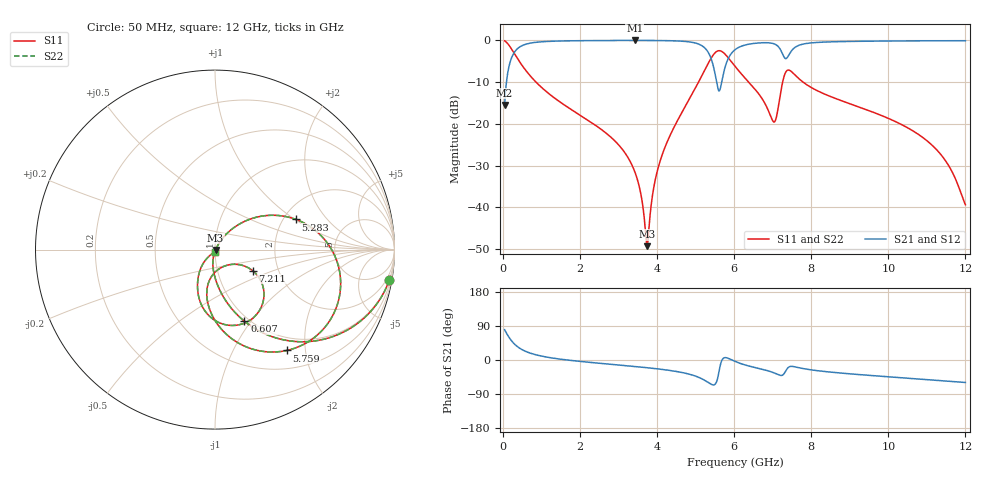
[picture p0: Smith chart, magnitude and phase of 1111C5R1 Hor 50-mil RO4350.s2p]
# GHz S MA R 50
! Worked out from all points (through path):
!   11951 points, 50 MHz to 12 GHz, reference 50 ohm
!   highest |S21| = -0.03 dB at 3.427 GHz (marker M1); lowest = -15.5 dB at 50 MHz (marker M2)
!   group delay of S21, straight-line fit = 16.3 ps
!   lowest |S11| = -49.3 dB at 3.745 GHz (marker M3), VSWR 1.01, Z = 50.3 - j0.136 ohm
!   |S11| at or under -10 dB: 864.7 MHz to 5.079 GHz (4.215 GHz wide, 142 % of centre); 6.381 GHz to 7.26 GHz (879.6 MHz wide, 12.9 % of centre); 7.79 GHz to end of sweep
!   |S22| runs from -49.3 to -0.1 dB; largest |S21 - S12| = 0
!   S11 on the Smith chart (normalised r, x): 50 MHz: 1, -11; 607 MHz: 0.95, -0.93; 5.283 GHz: 2.33, +1.02; 5.759 GHz: 0.78, -1.66; 7.211 GHz: 1.48, -0.37; 12 GHz: 1.00, -0.02
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0.05  0.9858 -10.0  0.1681 80.0  0.1681 80.0  0.9858 -10.0
0.238  0.7759 -40.4  0.6304 49.6  0.6304 49.6  0.7759 -40.4
0.607  0.432 -67.6  0.9011 22.3  0.9011 22.3  0.432 -67.6
2.042  0.1242 -93.4  0.9908 -4.1  0.9908 -4.1  0.1242 -93.4
2.956  0.05945 -100.9  0.9961 -12.7  0.9961 -12.7  0.05945 -100.9
3.427  0.02665 -101.5  0.9968 -17.1  0.9968 -17.1  0.02665 -101.5
3.579  0.01485 -97.2  0.9967 -18.6  0.9967 -18.6  0.01485 -97.2
3.745  0.003438 -23.2  0.9963 -20.3  0.9963 -20.3  0.003438 -23.2
4.034  0.03005 57.3  0.9946 -23.6  0.9946 -23.6  0.03005 57.3
4.844  0.1993 46.1  0.9579 -37.5  0.9579 -37.5  0.1993 46.1
5.283  0.4817 20.4  0.7726 -56.4  0.7726 -56.4  0.4817 20.4
5.601  0.7513 -28.2  0.25 -35.6  0.25 -35.6  0.7513 -28.2
5.759  0.6896 -54.6  0.4618 6.2  0.4618 6.2  0.6896 -54.6
6.025  0.4888 -81.0  0.7718 -3.7  0.7718 -3.7  0.4888 -81.0
6.492  0.2771 -99.2  0.916 -18.6  0.916 -18.6  0.2771 -99.2
7.019  0.1065 -72.1  0.9144 -33.3  0.9144 -33.3  0.1065 -72.1
7.211  0.2397 -29.2  0.7636 -40.8  0.7636 -40.8  0.2397 -29.2
7.447  0.4359 -75.7  0.6993 -17.4  0.6993 -17.4  0.4359 -75.7
8.017  0.2703 -110.0  0.9333 -26.3  0.9333 -26.3  0.2703 -110.0
10.009  0.116 -129.0  0.9819 -44.4  0.9819 -44.4  0.116 -129.0
11.285  0.04733 -131.6  0.9883 -53.9  0.9883 -53.9  0.04733 -131.6
12  0.01077 -79.8  0.9893 -59.3  0.9893 -59.3  0.01077 -79.8
